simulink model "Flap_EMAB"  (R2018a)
settings: Solver=ode45  StartTime=0.0  StopTime=0.4  RelTol=1e-3  EnableMultiTasking=on
InitFcn:
  | init
StopFcn:
  | pl
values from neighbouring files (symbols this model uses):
  Be = 25    [init.m]
  d2r = pi/180    (= 0.0174532925199)    [init.m]
  Ja = 2.0e-4    (= 0.0002)    [init.m]
  Je = 2.2    [init.m]
  Jm = 5.0e-5    (= 5e-05)    [init.m]
  Kdmp = 0.001    [init.m]
  Keff = 0.85    [init.m]
  Kgs = 400.0    (= 400)    [init.m]
  Ki = 5.0    (= 5)    [init.m]
  Kl = 12/Kli    (= 1800000)    [init.m]
  Kmfr = 0.03    [init.m]
  Kp = 140    [init.m]
  Kratlm = 0.1    [init.m]
  Krfb = 0.0005    [init.m]
  Kt = 12/Kti    (= 1674418.60465)    [init.m]
  Kv = 260    [init.m]
  Kw = 0    [init.m]
  Ngear = 10.2    [init.m]
  Nscrew = 0.0026    [init.m]
  R = 0.287    [init.m]    (also in lqr_des.m = diag(R))
  Vlim = 100    [init.m]
  Wmb = 1500    [init.m]
undefined symbols (not defined in the file or in its folder): coulomb

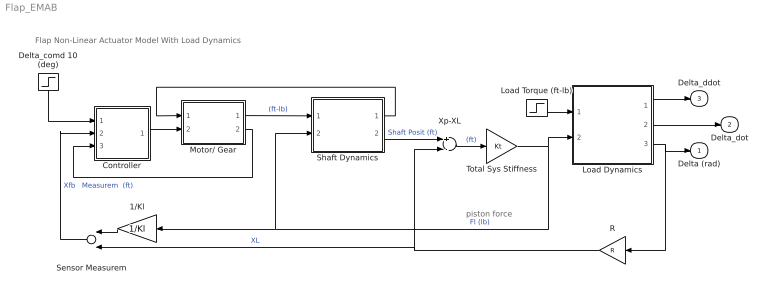
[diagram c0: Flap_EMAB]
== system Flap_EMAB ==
  note: piston force
  note: Flap Non-Linear Actuator Model With Load Dynamics
  1/Kl : Gain  Gain=1/Kl
  Controller : Subsystem
  Delta_comd 10 (deg) : Step  Time=0  After=10  SampleTime=0
  Load Dynamics : Subsystem
  Load Torque (ft-lb) : Step  Time=0  After=0  SampleTime=0
  Motor/ Gear : Subsystem
  R : Gain  Gain=R
  Sensor Measurem : Sum
  Shaft Dynamics : Subsystem
  Total Sys Stiffness : Gain  Gain=Kt
  Xp-XL : Sum  Inputs=+-
  Delta (rad) : Outport
  Delta_dot : Outport  Port=2
  Delta_ddot : Outport  Port=3
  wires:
  Shaft Dynamics/2(Xp) -> Xp-XL/1  "Shaft Posit (ft)"
  Xp-XL/1 -> Total Sys Stiffness/1  "(ft)"
  Total Sys Stiffness/1 -> 1/Kl/1, Shaft Dynamics/2(FL), Load Dynamics/2(FL)  "Fl (lb)"
  1/Kl/1 -> Sensor Measurem/1
  Controller/1(V) -> Motor/ Gear/2(Vin)
  Motor/ Gear/1(Tm) -> Shaft Dynamics/1(Tq-mot)  "(ft-lb)"
  Load Dynamics/1(Del_ddot) -> Delta_ddot/1
  Load Dynamics/3(Delta (rad)) -> Delta (rad)/1, R/1
  Load Dynamics/2(Delta_dot) -> Delta_dot/1
  Sensor Measurem/1 -> Controller/2(Xp-fb)  "Xfb   Measurem  (ft)"
  Shaft Dynamics/1(Xp-dot) -> Motor/ Gear/1(Xp-dot)
  R/1 -> Sensor Measurem/2, Xp-XL/2  "XL"
  Motor/ Gear/2(mr) -> Controller/3(rotor)
  Delta_comd 10 (deg)/1 -> Controller/1(delt-cmd)
  Load Torque (ft-lb)/1 -> Load Dynamics/1(TL)

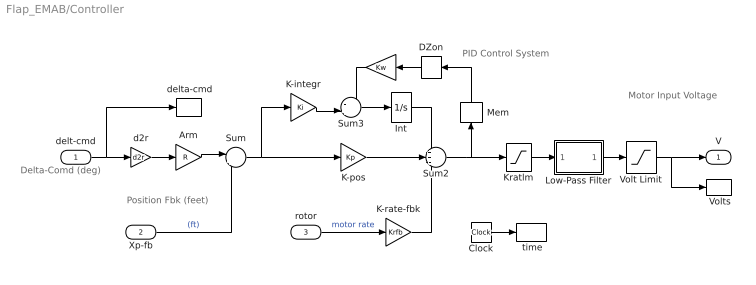
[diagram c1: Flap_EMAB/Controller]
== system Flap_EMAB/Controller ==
  note: PID Control System
  note: Motor Input Voltage
  note: Delta-Comd (deg)
  note: Position Fbk (feet)
  delt-cmd : Inport
  Xp-fb : Inport  Port=2
  rotor : Inport  Port=3
  " " : Gain  Gain=Kw
  " Volts" : ToWorkspace  VariableName=V  SampleTime=-1
  " delta-cmd" : ToWorkspace  VariableName=delc  SampleTime=-1
  " time" : ToWorkspace  VariableName=time  SampleTime=-1
  Arm : Gain  Gain=R
  Clock : Clock
  DZon : DeadZone  LowerValue=-Vlim  UpperValue=Vlim
  Int : Integrator  LimitOutput=on  UpperSaturationLimit=1  LowerSaturationLimit=-1
  K-integr : Gain  Gain=Ki
  K-pos : Gain  Gain=Kp
  K-rate-fbk : Gain  Gain=Krfb
  Kratlm : Saturate  UpperLimit=Kratlm  LowerLimit=-Kratlm
  Low-Pass Filter : Subsystem
  Mem : Memory
  Sum : Sum  Inputs=|+-
  Sum2 : Sum  Inputs=++-
  Sum3 : Sum  Inputs=-+|
  Volt Limit : Saturate  UpperLimit=Vlim  LowerLimit=-Vlim
  d2r : Gain  Gain=d2r
  V : Outport
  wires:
  delt-cmd/1 -> " delta-cmd"/1, d2r/1
  Xp-fb/1 -> Sum/2  "(ft)"
  Sum/1 -> K-pos/1, K-integr/1
  rotor/1 -> K-rate-fbk/1  "motor rate"
  Sum2/1 -> Kratlm/1, Mem/1
  K-pos/1 -> Sum2/2
  Volt Limit/1 -> V/1, " Volts"/1
  Clock/1 -> " time"/1
  K-integr/1 -> Sum3/2
  Sum3/1 -> Int/1
  Int/1 -> Sum2/1
  DZon/1 -> " "/1
  Mem/1 -> DZon/1
  K-rate-fbk/1 -> Sum2/3
  d2r/1 -> Arm/1
  Arm/1 -> Sum/1
  Kratlm/1 -> Low-Pass Filter/1(in)
  " "/1 -> Sum3/1
  Low-Pass Filter/1(ou) -> Volt Limit/1

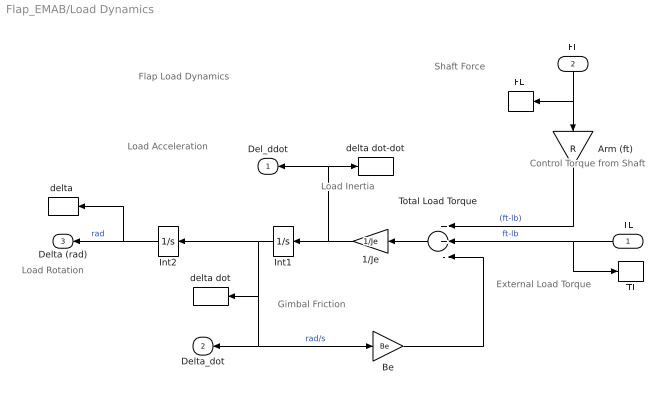
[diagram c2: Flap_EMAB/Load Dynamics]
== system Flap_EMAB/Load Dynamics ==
  note: Flap Load Dynamics
  note: Load Rotation
  note: Load Inertia
  note: Gimbal Friction
  note: Load Acceleration
  note: External Load Torque
  note: Control Torque from Shaft
  note: Shaft Force
  TL : Inport
  FL : Inport  Port=2
  1/Je : Gain  Gain=1/Je
  Arm (ft) : Gain  Gain=R
  Be : Gain  Gain=Be
  "FL " : ToWorkspace  VariableName=FL  SampleTime=-1
  Int1 : Integrator
  Int2 : Integrator
  Tl : ToWorkspace  VariableName=TL  SampleTime=-1
  Total Load Torque : Sum  Inputs=++-
  delta dot : ToWorkspace  VariableName=deldot  SampleTime=-1
  delta dot-dot : ToWorkspace  VariableName=deldd  SampleTime=-1
  "delta " : ToWorkspace  VariableName=delta  SampleTime=-1
  Del_ddot : Outport
  Delta_dot : Outport  Port=2
  Delta (rad) : Outport  Port=3
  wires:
  Arm (ft)/1 -> Total Load Torque/1  "(ft-lb)"
  Be/1 -> Total Load Torque/3
  Total Load Torque/1 -> 1/Je/1
  Int2/1 -> Delta (rad)/1, "delta "/1  "rad"
  TL/1 -> Total Load Torque/2, Tl/1  "ft-lb"
  FL/1 -> Arm (ft)/1, "FL "/1
  Int1/1 -> Int2/1, Be/1, Delta_dot/1, delta dot/1  "rad/s"
  1/Je/1 -> Int1/1, Del_ddot/1, delta dot-dot/1

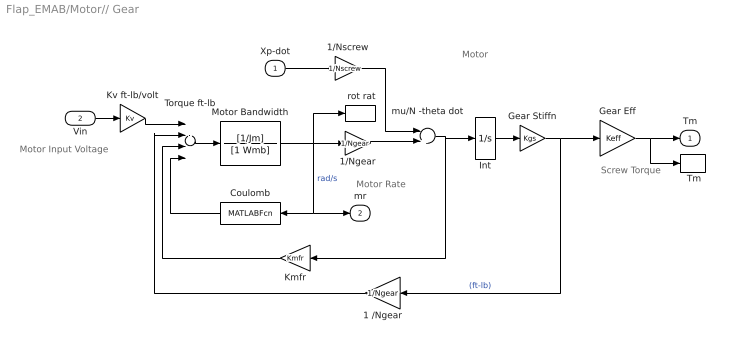
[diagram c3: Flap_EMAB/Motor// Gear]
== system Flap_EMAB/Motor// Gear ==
  note: Motor
  note: Motor Input Voltage
  note: Screw Torque
  note: Motor Rate
  Xp-dot : Inport
  Vin : Inport  Port=2
  " Tm" : ToWorkspace  VariableName=Tm  SampleTime=-1
  " rot rat" : ToWorkspace  VariableName=mrat  SampleTime=-1
  1 /Ngear : Gain  Gain=1/Ngear
  1/Ngear : Gain  Gain=1/Ngear
  1/Nscrew : Gain  Gain=1/Nscrew
  Coulomb : MATLABFcn  MATLABFcn=coulomb(0.002, u(1) )
  Gear Eff : Gain  Gain=Keff
  Gear Stiffn : Gain  Gain=Kgs
  Int : Integrator  LimitOutput=on  UpperSaturationLimit=0.4  LowerSaturationLimit=-0.4
  Kmfr : Gain  Gain=Kmfr
  Kv ft-lb/volt : Gain  Gain=Kv
  Motor Bandwidth : TransferFcn  Numerator=[1/Jm]  Denominator=[1 Wmb]
  Torque ft-lb : Sum  Inputs=+---
  mu/N -theta dot : Sum  Inputs=-+
  Tm : Outport
  mr : Outport  Port=2
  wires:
  mu/N -theta dot/1 -> Int/1, Kmfr/1
  Torque ft-lb/1 -> Motor Bandwidth/1
  1 /Ngear/1 -> Torque ft-lb/2
  Motor Bandwidth/1 -> 1/Ngear/1, " rot rat"/1, mr/1, Coulomb/1  "rad/s"
  1/Ngear/1 -> mu/N -theta dot/2
  Gear Stiffn/1 -> 1 /Ngear/1, Gear Eff/1  "(ft-lb)"
  Xp-dot/1 -> 1/Nscrew/1
  Vin/1 -> Kv ft-lb/volt/1
  Gear Eff/1 -> Tm/1, " Tm"/1
  Kv ft-lb/volt/1 -> Torque ft-lb/1
  1/Nscrew/1 -> mu/N -theta dot/1
  Kmfr/1 -> Torque ft-lb/3
  Int/1 -> Gear Stiffn/1
  Coulomb/1 -> Torque ft-lb/4

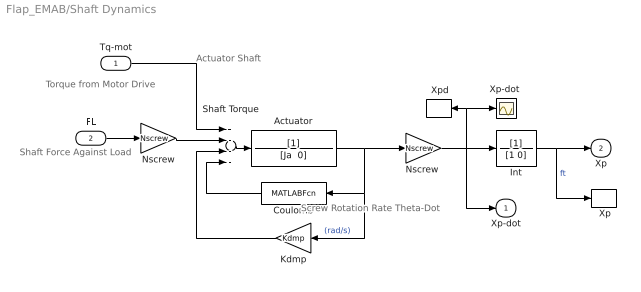
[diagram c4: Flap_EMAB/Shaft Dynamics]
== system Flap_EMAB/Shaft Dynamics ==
  note: Actuator Shaft
  note: Torque from Motor Drive
  note: Shaft Force Against Load
  note: Screw Rotation Rate Theta-Dot
  Tq-mot : Inport
  FL : Inport  Port=2
  " Xp" : ToWorkspace  VariableName=Xp  SampleTime=-1
  " Xpd" : ToWorkspace  VariableName=Xpd  SampleTime=-1
  Actuator : TransferFcn  Denominator="[Ja  0]"
  Coulomb : MATLABFcn  MATLABFcn=coulomb(0.05, u(1) )
  Int : TransferFcn  Denominator=[1 0]
  Kdmp : Gain  Gain=Kdmp
  Nscrew : Gain  Gain=Nscrew
  "Nscrew " : Gain  Gain=Nscrew
  Shaft Torque : Sum  Inputs=+---
  "Xp-dot " : Scope
  Xp-dot : Outport
  Xp : Outport  Port=2
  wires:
  Actuator/1 -> Kdmp/1, Coulomb/1, "Nscrew "/1  "(rad/s)"
  Shaft Torque/1 -> Actuator/1
  Tq-mot/1 -> Shaft Torque/1
  Int/1 -> Xp/1, " Xp"/1  "ft"
  FL/1 -> Nscrew/1
  Nscrew/1 -> Shaft Torque/2
  "Nscrew "/1 -> Int/1, "Xp-dot "/1, " Xpd"/1, Xp-dot/1
  Kdmp/1 -> Shaft Torque/3
  Coulomb/1 -> Shaft Torque/4

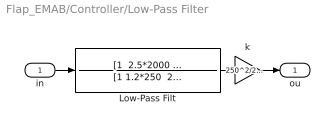
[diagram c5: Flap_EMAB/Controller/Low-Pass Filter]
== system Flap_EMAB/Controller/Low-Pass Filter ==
  in : Inport
  Low-Pass Filt : TransferFcn  Numerator="[1  2.5*2000  2000^2]"  Denominator="[1 1.2*250  250^2]"
  k : Gain  Gain=250^2/2000^2
  ou : Outport
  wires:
  Low-Pass Filt/1 -> k/1
  in/1 -> Low-Pass Filt/1
  k/1 -> ou/1
